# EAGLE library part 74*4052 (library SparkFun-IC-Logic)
Dual 4:1 Analog Mux Dual four-channel analog MULTIPLEXER / DEMULTIPLEXER SparkFun Products SparkFun Vernier Interface Shield (DEV-12858)
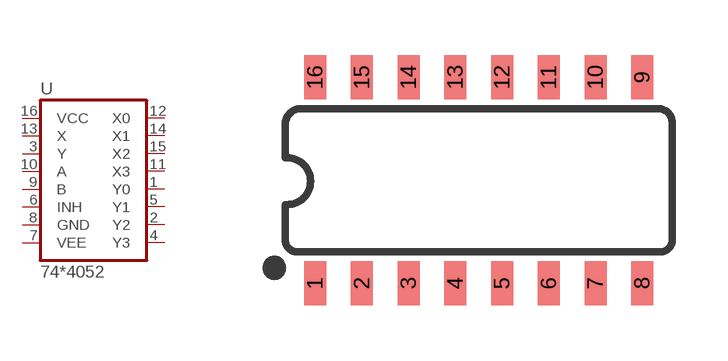
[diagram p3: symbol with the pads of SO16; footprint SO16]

Designator prefix U

## 74HC4052D (PROD_ID: IC-13103; VALUE: 74HC4052D)  [SO16]
1  Y0
2  Y2
3  Y
4  Y3
5  Y1
6  INH  in
7  VEE  pwr
8  GND  pwr
9  B  in
10  A  in
11  X3
12  X0
13  X
14  X1
15  X2
16  VCC  pwr

## Footprint SO16 (pad centres in mm)
SOIC, 0.15 inch width
smd 0.6 x 1.2: 1 -4.445,-2.8; 2 -3.175,-2.8; 3 -1.905,-2.8; 4 -0.635,-2.8; 5 0.635,-2.8; 6 1.905,-2.8; 7 3.175,-2.8; 8 4.445,-2.8; 9 4.445,2.8; 10 3.175,2.8; 11 1.905,2.8; 12 0.635,2.8; 13 -0.635,2.8; 14 -1.905,2.8; 15 -3.175,2.8; 16 -4.445,2.8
